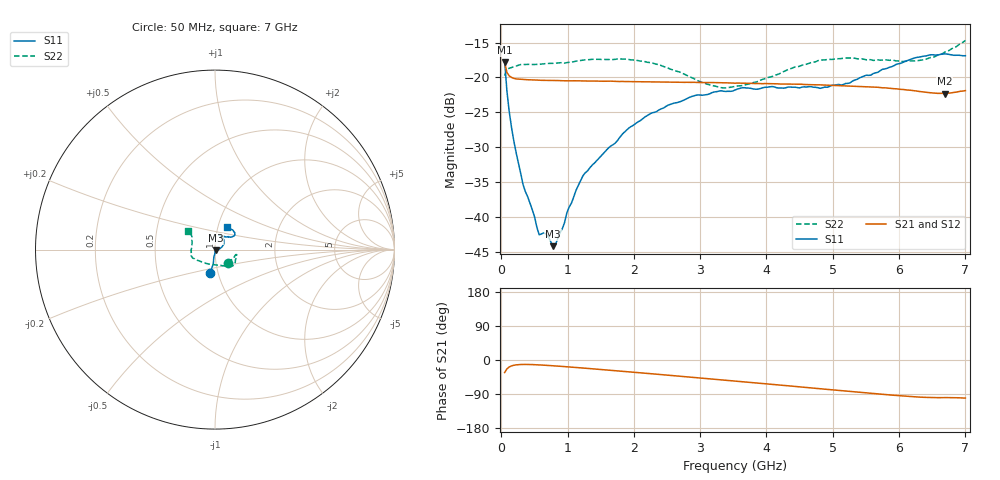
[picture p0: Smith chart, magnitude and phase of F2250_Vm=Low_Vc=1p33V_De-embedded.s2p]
! Integrated Device Technology
! Corporate Headquarters
! 6024 Silver Creek Valley Road
! San Jose, CA 95138  USA
! Phone:  1-408-284-8200
! Toll Free:  1-800-223-1366
! Webpage:  http://www.idt.com/
! Timing and RF Division
! 515 Groton Road, Suite 102
! Westford, MA 01886-6024
! Device:  F2250
! Description: Voltage Variable RF Attenuator
! Frequency:  50.0 -  6000.00 MHz
! Package:  3x3 mm Thin QFN Plastic Package: 16 pin
! Ports:  2 RF, 3 DC
!  Pin  1  = GND
!  Pin  2  = NC
!  Pin  3  = RF1  = Port 1
!  Pin  4  = NC
!  Pin  5  = GND
!  Pin  6  = GND
!  Pin  7  = GND
!  Pin  8  = GND
!  Pin  9  = NC
!  Pin 10  = RF2  = Port 2
!  Pin 11  = NC
!  Pin 12  = GND
!  Pin 13  = GND
!  Pin 14  = VCNTRL
!  Pin 15  = VDD
!  Pin 16  = VMODE
! Vcntrl:  1.330 Volts
! Vmode:  +0.000 Volts
! Vdd:  +3.30  Volts
! Current:  1.192 mA
! Data:  The device was measured on a the F2250 evaluation board which has
!  individual transmission lines to the RF pins.  Data was collected
!  using a calibrated network analyzer.  The evaluation board was
!  de-embedded using a TRL calibration technique.
!  The reference plane is the edge of the package pin.
! Misc:  SN 10
!  Action Tracker AT0258
! Date Measured:  2014-11-26
! Date:  2015-10-15  MJV
! Note:
!  Integrated Device Technology supplies this data as a sample of measured
!  data at the package pin for this product.  Your particular data for this
!  product may vary.
!  Data was taken at 25 degrees C.
!  Integrated Device Technology reserves the right to change this data at anytime.
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# GHz S dB R 50
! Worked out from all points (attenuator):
!   201 points, 50 MHz to 7 GHz, reference 50 ohm
!   highest |S21| = -17.83 dB at 50 MHz (marker M1); lowest = -22.3 dB at 6.687 GHz (marker M2)
!   lowest |S11| = -44.2 dB at 779.8 MHz (marker M3), VSWR 1.01, Z = 50.5 - j0.345 ohm
!   |S11| at or under -10 dB: start of sweep to end of sweep
!   |S22| runs from -21.5 to -14.7 dB; largest |S21 - S12| = 0.00035
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0.05  -17.61 -101.8  -17.83 -33.1  -17.83 -33.1  -19.74 -46.6
0.08475  -21.93 -96.9  -19.29 -23.4  -19.29 -23.4  -18.85 -23.4
0.15425  -27.15 -98.6  -19.99 -15.6  -20.00 -15.6  -18.59 -14.3
0.328  -35.32 -90.3  -20.29 -11.7  -20.29 -11.7  -18.13 -13.0
0.467  -38.93 -87.1  -20.36 -12.1  -20.38 -12.1  -18.15 -14.7
0.57125  -42.53 -68.2  -20.39 -12.9  -20.40 -12.9  -18.12 -17.4
0.6755  -42.41 -55.4  -20.42 -14.0  -20.41 -14.0  -18.01 -19.7
0.77975  -44.16 -33.5  -20.44 -15.2  -20.43 -15.2  -17.98 -22.4
0.8145  -43.99 -27.0  -20.45 -15.6  -20.43 -15.6  -17.95 -23.4
0.91875  -41.69 -14.2  -20.47 -16.9  -20.46 -16.9  -17.87 -26.1
0.98825  -39.41 -19.0  -20.47 -17.8  -20.48 -17.8  -17.88 -27.3
1.2315  -34.08 0.5  -20.48 -21.1  -20.48 -21.2  -17.50 -32.2
1.9265  -27.22 22.6  -20.59 -31.3  -20.58 -31.3  -17.44 -42.1
2.37825  -24.65 33.2  -20.64 -38.0  -20.63 -38.0  -18.17 -49.5
3.14275  -22.35 54.9  -20.73 -49.7  -20.72 -49.8  -21.07 -79.3
3.525  -21.80 65.6  -20.82 -55.6  -20.81 -55.7  -21.29 -105.9
4.7065  -21.40 68.9  -21.04 -74.2  -21.04 -74.2  -17.83 -157.2
5.22775  -20.85 52.2  -21.22 -82.4  -21.20 -82.5  -17.22 -166.3
5.85325  -18.55 36.9  -21.56 -92.1  -21.56 -92.2  -17.55 -178.8
6.33975  -17.01 38.5  -22.05 -98.1  -22.04 -98.3  -17.51 163.4
6.68725  -16.62 47.0  -22.31 -99.2  -22.30 -99.3  -16.37 149.2
7  -16.89 62.7  -21.88 -100.4  -21.87 -100.5  -14.70 145.5
